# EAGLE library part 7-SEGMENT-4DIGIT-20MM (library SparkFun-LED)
4 Digit 7 Segment Display This is a part for the 4-Digit 7-segment LEDs from Young Sun. Different from the Digikey LEDs, all 16 pins are used. The LONGPADS Variant is used for a test jig, but you may like it because there is more pad to solder to. If you are concerned about routing space, the standard works just fine though. Datasheets: Red Yellow Green Blue White SparkFun Products Raw Components 7-Segment Display - 20mm (Red) (COM-11405) 7-Segment Display - 20mm (Yellow) (COM-11406) 7-Segment Display - 20mm (Green) (COM-11407) 7-Segment Display - 20mm (Blue) (COM-11408) 7-Segment Display - 20mm (White) (COM-11409) Serial Controlled SparkFun OpenSegment Serial Display - 20mm (Red) (COM-11644) SparkFun OpenSegment Serial Display - 20mm (Yellow) (COM-11645) SparkFun OpenSegment Serial Display - 20mm (Green) (COM-11646) SparkFun OpenSegment Serial Display - 20mm (Blue) (COM-11647) SparkFun OpenSegment Serial Display - 20mm (White) (COM-11648) Other SparkFun OpenSegment Shield (DEV-13190)
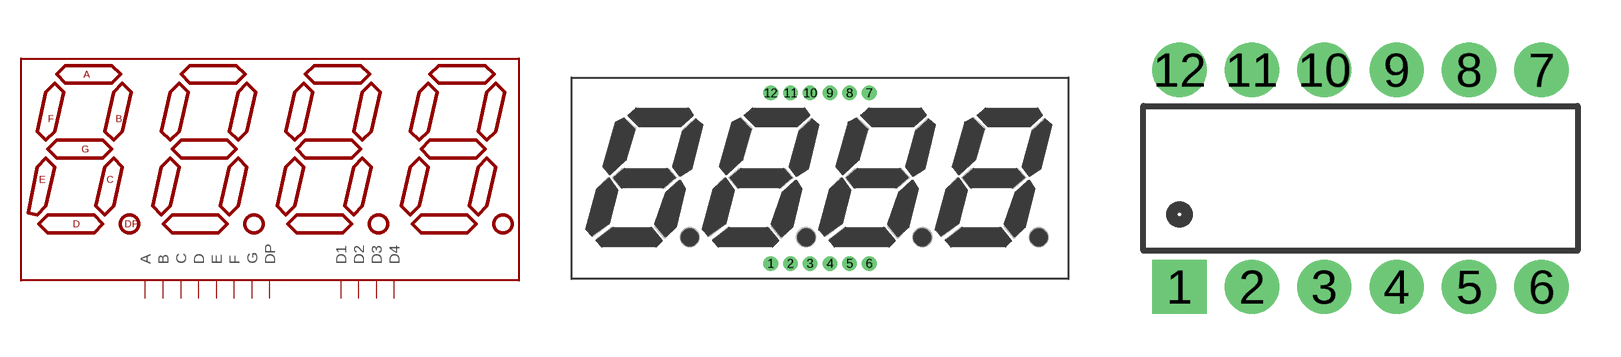
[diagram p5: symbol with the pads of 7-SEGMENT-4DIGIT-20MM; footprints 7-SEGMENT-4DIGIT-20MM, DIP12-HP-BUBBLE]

Designator prefix DISP

## 7-SEGMENT-4DIGIT-20MM-RED (PROD_ID: COMP-11449; VALUE: ATA8041ARBJ)  [7-SEGMENT-4DIGIT-20MM]
1  E
2  D
3  DP
4  C
5  G
6  D4
7  B
8  D3
9  D2
10  F
11  A
12  D1

## 7-SEGMENT-4DIGIT-20MM-HP-BUBBLE (STOREFRONT: COM-12710)  [DIP12-HP-BUBBLE]
1  D1
2  E
3  C
4  D3
5  DP
6  D4
7  G
8  D
9  F
10  D2
11  B
12  A

## 7-SEGMENT-4DIGIT-20MM-YELLOW (PROD_ID: COMP-11448; VALUE: ATA8041AY)  [7-SEGMENT-4DIGIT-20MM]
Pads as for 7-SEGMENT-4DIGIT-20MM

## 7-SEGMENT-4DIGIT-20MM-GREEN (PROD_ID: COMP-11447; VALUE: ATA8041AG)  [7-SEGMENT-4DIGIT-20MM]
Pads as for 7-SEGMENT-4DIGIT-20MM

## 7-SEGMENT-4DIGIT-20MM-BLUE (PROD_ID: COMP-11446; VALUE: ATA8041AB)  [7-SEGMENT-4DIGIT-20MM]
Pads as for 7-SEGMENT-4DIGIT-20MM

## 7-SEGMENT-4DIGIT-20MM-WHITE (PROD_ID: COMP-11445; VALUE: ATA8041AW)  [7-SEGMENT-4DIGIT-20MM]
Pads as for 7-SEGMENT-4DIGIT-20MM

## Footprint 7-SEGMENT-4DIGIT-20MM (pad centres in mm)
drill 0.9 pad 1.88: 1 -6.35,-10.998; 2 -3.81,-10.998; 3 -1.27,-10.998; 4 1.27,-10.998; 5 3.81,-10.998; 6 6.35,-10.998; 7 6.35,10.998; 8 3.81,10.998; 9 1.27,10.998; 10 -1.27,10.998; 11 -3.81,10.998; 12 -6.35,10.998

## Footprint DIP12-HP-BUBBLE (pad centres in mm)
drill 0.864 pad 1.905 square: 1 -6.35,-3.81
drill 0.864 pad 1.905: 2 -3.81,-3.81; 3 -1.27,-3.81; 4 1.27,-3.81; 5 3.81,-3.81; 6 6.35,-3.81; 7 6.35,3.81; 8 3.81,3.81; 9 1.27,3.81; 10 -1.27,3.81; 11 -3.81,3.81; 12 -6.35,3.81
